PROGRAM MAIN
VAR
	//指定行列
	Columnneo					: INT := 2;   //列数
	Columnname				: STRING := 'Name';  //列头名
	Rowneo						: INT := 3;   //行数
	RowID							: INT := 800; 	//行头名
	Rownumber				: INT := 5; //指定单元格行数
	Columnnumber			: INT := 4; //指定单元格列数
	
	// 读取结果
	ReadByColumnneo			: ARRAY[0..40] OF STRING;   //指定列读取结果
	ReadByColumnname		: ARRAY[0..40] OF STRING;  //指定列头名读取结果
	ReadByRowname             	: STRING(400);	  //指定行头名读取结果
	ReadByRowneo					: STRING;  //指定行数读取结果
	ReadByiloc							: STRING;  // 指定单元格读取结果
	
	
	//字符串分割
	SeparatorRowneo				: STRING := ',';
	SplitRowneoString			: ARRAY[1..cMaxRowneo] OF STRING(255);
	ResultSplitRowneo			: BOOL;
	i_Rowneo							: UDINT;
	
	SeparatorRowname			: STRING := ',';
	SplitRownameString			: ARRAY[1..cMaxRowname] OF STRING(400);
	ResultSplitRowname			: BOOL;
	i_Rowname							: UDINT;
END_VAR

VAR CONSTANT
	cMaxRowneo							: UDINT := 11;
	cMaxRowname						: UDINT := 10;
END_VAR

//按行读取的字符串处理
SplitRowneoString[1] := ReadByRowneo;
FOR i_Rowneo:=1 TO cMaxRowneo-1 DO
   		ResultSplitRowneo := FindAndSplit( pSeparator     := ADR(SeparatorRowneo),  pSrcString := ADR(SplitRowneoString[i_Rowneo]), 
                                  pLeftString    := ADR(SplitRowneoString[i_Rowneo]),   nLeftSize  := SIZEOF(SplitRowneoString[i_Rowneo]), 
                                  pRightString   := ADR(SplitRowneoString[i_Rowneo+1]), nRightSize := SIZEOF(SplitRowneoString[i_Rowneo+1]),
                                  bSearchFromRight := FALSE );
  		IF NOT ResultSplitRowneo THEN
       				  EXIT;
        END_IF
END_FOR

//按行头读取的字符串处理
SplitRownameString[1] := ReadByRowname;
FOR i_Rowname:=1 TO cMaxRowname-1 DO
   		ResultSplitRowname := FindAndSplit( pSeparator     := ADR(SeparatorRowname),  pSrcString := ADR(SplitRownameString[i_Rowname]), 
                                  pLeftString    := ADR(SplitRownameString[i_Rowname]),   nLeftSize  := SIZEOF(SplitRownameString[i_Rowname]), 
                                  pRightString   := ADR(SplitRownameString[i_Rowname+1]), nRightSize := SIZEOF(SplitRownameString[i_Rowname+1]),
                                  bSearchFromRight := false );
  		IF NOT ResultSplitRowname THEN
       				  EXIT;
        END_IF
END_FOR

END_PROGRAM
